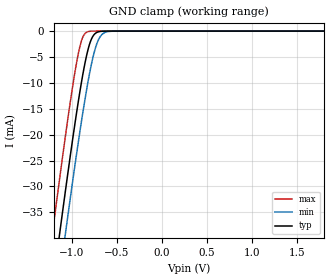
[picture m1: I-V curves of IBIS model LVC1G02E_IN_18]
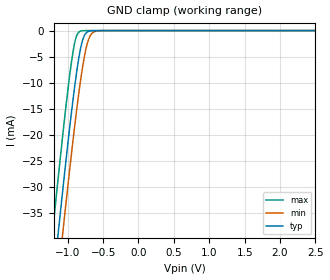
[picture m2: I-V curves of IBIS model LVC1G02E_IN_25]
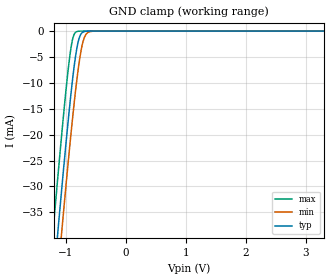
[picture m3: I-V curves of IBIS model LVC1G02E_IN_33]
| TEXAS INSTRUMENTS INCORPORATED
| Standard Linear and Logic Group
| IBIS Model of SN74LVC1G02
| SINGLE 2-INPUT POSITIVE-NOR GATE
| This file contains package information for the following:
|  SOT 5-pin (DBV) package as [Component] LVC1G02E_DBV
|  SOT 5-pin (DCK) package as [Component] LVC1G02E_DCK
|  USON 6-pin (DRY) package as [Component] LVC1G02_DRY
| This device can be powered at the following Vccs:
|  1.8 volt Vcc
|  2.5 volt Vcc
|  3.3 volt Vcc
|  5 volt Vcc
| This file provides unique models under the [Model Selector] for each Vcc.
| For operation at a specific Vcc, select the appropriate model after each
| [Model Selector] keyword.
[IBIS Ver]   4.1
[Comment char]  |_char
[File Name]   sn74lvc1g02.ibs
[File Rev]   1.2 | e_die
[Date]   April 24, 2013
[Source]   Data created from TI-SPICE simulations at TI-SLL.
[Notes]   Revision History:
   Rev 1.2. Added package component LVC1G02_DRY
   - Due to the fact that the Device is 5.5-V Input tolarent,
   the pulldown model has some Non-Monotonic Warnings.
   - Power clamp data deleted as there is no power-clamp diode.
[Disclaimer]  This model is designed as an aid for customers of Texas Instruments
 TI and its licensors and suppliers make no warranties, either expressed
 or implied, with respect to this  model, including the warranties of
 merchantability or fitness for a particular purpose.
 The model is provided solely on an "as is" basis. The entire risk as to
 its quality and performance is with the customer.
[Copyright] (C)Copyright 2013 Texas Instruments Incorporated.
   All rights reserved.
| Component LVC1G02E_DBV 5-pin SOT
[Component]   LVC1G02E_DBV
[Manufacturer]   Texas Instruments, Inc.
[Package]
|   typ   min   max
R_pkg   2.500e-02   2.100e-02   2.900e-02
L_pkg   1.529e-09   1.312e-09   1.906e-09
C_pkg   1.560e-13   1.100e-13   2.400e-13
[Pin]   signal_name   model_name   R_pin   L_pin   C_pin
1   A1   LVC1G02E_IN   2.100e-02   1.511e-09   1.440e-13
2   B1   LVC1G02E_IN   2.300e-02   1.312e-09   1.380e-13
3   GND   GND   2.900e-02   1.906e-09   2.400e-13
4   Y1   LVC1G02E_OUT   2.600e-02   1.541e-09   1.500e-13
5   VCC   POWER   2.500e-02   1.374e-09   1.100e-13
| Component LVC1G02E_DCK 5-pin SOT
[Component]   LVC1G02E_DCK
[Manufacturer]   Texas Instruments, Inc.
[Package]
|   typ   min   max
R_pkg   2.000e-02   1.700e-02   2.500e-02
L_pkg   9.980e-10   8.810e-10   1.069e-09
C_pkg   1.460e-13   1.180e-13   2.050e-13
[Pin]   signal_name   model_name   R_pin   L_pin   C_pin
1   A1   LVC1G02E_IN   1.900e-02   1.069e-09   1.620e-13
2   B1   LVC1G02E_IN   1.800e-02   8.810e-10   1.210e-13
3   GND   GND   1.700e-02   1.031e-09   2.050e-13
4   Y1   LVC1G02E_OUT   2.000e-02   9.600e-10   1.240e-13
5   VCC   POWER   2.500e-02   1.049e-09   1.180e-13
| Component LVC1G02_DRY 6-pin USON
[Component]   LVC1G02_DRY
[Manufacturer]   Texas Instruments, Inc.
[Package]
|   typ   min   max
R_pkg   0.04988   0.00103   0.05683
L_pkg   0.40631n   0.01445n   0.47858n
C_pkg   0.10742p   0.07652p   0.11194p
[Pin]   signal_name   model_name   R_pin   L_pin   C_pin
1   A   LVC1G02E_IN   0.05683   0.47858n   0.11194p
2   A   LVC1G02E_IN   0.04686   0.38124n   0.10769p
3   GND   GND   0.05415   0.45213n   0.10986p
4   Y   LVC1G02E_OUT   0.05132   0.42056n   0.10715p
5   NC   NC   0.00103   0.01445n   0.07652p
6   VCC   POWER   0.04843   0.39205n   0.10505p
| Model LVC1G02E_IN
[Model Selector]   LVC1G02E_IN
LVC1G02E_IN_18   1.8 volt Vcc
LVC1G02E_IN_25   2.5 volt Vcc
LVC1G02E_IN_33   3.3 volt Vcc
LVC1G02E_IN_50   5 volt Vcc
| Model LVC1G02E_OUT
[Model Selector]   LVC1G02E_OUT
LVC1G02E_OUT_18   1.8 volt Vcc
LVC1G02E_OUT_25   2.5 volt Vcc
LVC1G02E_OUT_33   3.3 volt Vcc
LVC1G02E_OUT_50   5 volt Vcc
| Models and submodels in the file (8): LVC1G02E_IN_18 (Input), LVC1G02E_IN_25 (Input), LVC1G02E_IN_33 (Input), LVC1G02E_IN_50 (Input), LVC1G02E_OUT_18 (Output), LVC1G02E_OUT_25 (Output), LVC1G02E_OUT_33 (Output), LVC1G02E_OUT_50 (Output)
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[Model]   LVC1G02E_IN_18
Model_type  Input
Vinl=0.5775
Vinh=1.2675
| variable   typ   min   max
C_comp   3.12pF   2.52pF   4.24pF
[Temperature Range]   40   100   -40
| Ambient temperature   25   85   -40
[Voltage range]   1.8   1.65   1.95
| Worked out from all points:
|   GND clamp passes 1 mA (typ) near -0.77 V on its own axis
[GND Clamp]
| LVC1G02E_IN_18
|   Voltage   I(typ)   I(min)   I(max)
-5.5V     -655.2mA   -662.2mA   -646.6mA
-1.215V   -49.6mA    -57.88mA   -38.96mA
-1.135V   -39.07mA   -47.36mA   -28.42mA
-1.075V   -31.35mA   -39.6mA    -20.75mA
-1.055V   -28.82mA   -37.05mA   -18.27mA
-955mV    -16.68mA   -24.66mA   -6.874mA
-885mV    -9.098mA   -16.55mA   -1.486mA
-825mV    -3.922mA   -10.26mA   -137.1uA
-780mV    -1.472mA   -6.227mA   -17.15uA
-715mV    -205.4uA   -2.128mA   -808.5nA
-650mV    -22.01uA   -443.9uA   -37.93nA
1.8V      3.326pA    6.142pA    3.026pA
[Model]   LVC1G02E_IN_25
Model_type  Input
Vinl=0.7
Vinh=1.7
| variable   typ   min   max
C_comp   3.14pF   2.51pF   4.31pF
[Temperature Range]   40   100   -40
| Ambient temperature   25   85   -40
[Voltage range]   2.5   2.3   2.7
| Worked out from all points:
|   GND clamp passes 1 mA (typ) near -0.77 V on its own axis
[GND Clamp]
| LVC1G02E_IN_25
|   Voltage   I(typ)   I(min)   I(max)
-5.5V     -655.2mA   -662.2mA   -646.6mA
-1.215V   -49.6mA    -57.88mA   -38.96mA
-1.14V    -39.72mA   -48.01mA   -29.07mA
-1.12V    -37.12mA   -45.41mA   -26.48mA
-1.08V    -31.98mA   -40.25mA   -21.38mA
-1.06V    -29.44mA   -37.69mA   -18.89mA
-960mV    -17.26mA   -25.26mA   -7.377mA
-890mV    -9.597mA   -17.1mA    -1.734mA
-785mV    -1.671mA   -6.635mA   -21.67uA
-720mV    -242.5uA   -2.354mA   -1.023uA
-650mV    -22.01uA   -443.9uA   -37.93nA
2.5V      4.713pA    7.577pA    4.389pA
[Model]   LVC1G02E_IN_33
Model_type  Input
Vinl=0.8
Vinh=2.0
| variable   typ   min   max
C_comp   3.16pF   2.51pF   4.43pF
[Temperature Range]   40   100   -40
| Ambient temperature   25   85   -40
[Voltage range]   3.3   3   3.6
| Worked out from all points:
|   GND clamp passes 1 mA (typ) near -0.77 V on its own axis
[GND Clamp]
| LVC1G02E_IN_33
|   Voltage   I(typ)   I(min)   I(max)
-5.5V     -655.2mA   -662.2mA   -646.6mA
-1.225V   -50.93mA   -59.21mA   -40.3mA
-1.145V   -40.37mA   -48.66mA   -29.72mA
-1.12V    -37.12mA   -45.41mA   -26.48mA
-1.08V    -31.98mA   -40.25mA   -21.38mA
-1.06V    -29.44mA   -37.69mA   -18.89mA
-965mV    -17.84mA   -25.87mA   -7.89mA
-885mV    -9.098mA   -16.55mA   -1.486mA
-780mV    -1.472mA   -6.227mA   -17.15uA
-715mV    -205.4uA   -2.128mA   -808.5nA
-640mV    -15.53uA   -338.1uA   -23.69nA
3.3V      6.304pA    9.258pA    5.93pA
